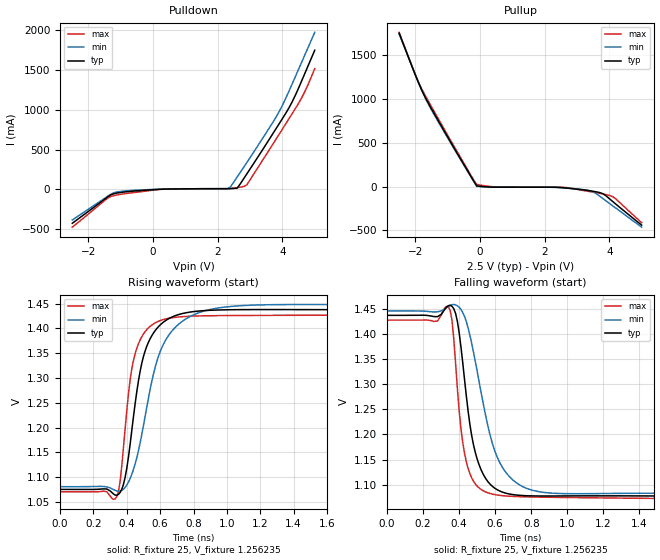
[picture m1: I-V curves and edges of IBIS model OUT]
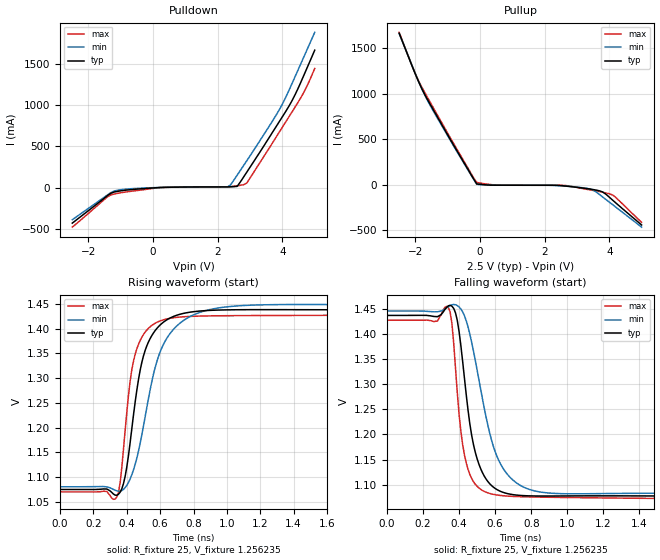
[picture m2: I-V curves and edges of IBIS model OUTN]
|   IBIS File of SG2520VGN D
|   LVDS, Vcc=2.5V, Io=7mA, fo>212.5MHz
[IBIS Ver]   3.2
[File Name]   sg2520vgn_hf_7m_25v.ibs
[File Rev]   1.0
[Date]   July 30, 2020
[Source]
Fairchild Ensigna Lab's Method
[Notes]
Created by Minoru Kozaki
[Disclaimer]
Seiko Epson Corporation makes no warranty with respect to the
information contained herein.
[Copyright]
Copyright(C) 2020, Seiko Epson Corporation. All rights reserved.
|   Component
[Component]   SG2520VGN
[Manufacturer]  Seiko Epson Corporation
[Package]
R_pkg   17.7m   NA   NA
L_pkg   235p   NA   NA
C_pkg   208f   NA   NA
[Pin]   signal_name   model_name   R_pin   L_pin   C_pin
1   OE/ST   NC
2   NC   NC
3   GND   GND
4   OUT   OUT   17.7m   235p   208f
5   OUTN   OUTN   10.4m   129p   221f
6   VCC   POWER
[Diff Pin] inv_pin  vdiff  tdelay_typ
4   5   0   0
| Models and submodels in the file (2): OUT (Output), OUTN (Output)
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|   Model OUT
[Model]   OUT
Model_type   Output
Polarity   Non-Inverting
Vref = 1.25
Vmeas = 1.25
Rref = 25
Cref = 0
C_comp   4.5p   4.5p   4.5p
[Temperature Range]   25   105   -40
[Voltage Range]   2.5   2.25   2.75
[Pullup Reference]   2.5   2.25   2.75
[Pulldown Reference]   0   0   0
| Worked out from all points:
|   slope of the pulldown table from 0 to 0.375 V, typ, clamps not added: 51.8 ohm
|   slope of the pullup table from 0 to 0.375 V, typ, clamps not added: 39.7 ohm
|   falling waveform, R_fixture 25, V_fixture 1.256235: 20-80 % time 89.9ps typ, 138ps min, 65.2ps max; typ from 1.44 V to 1.08 V
|   rising waveform, R_fixture 25, V_fixture 1.256235: 20-80 % time 108ps typ, 157ps min, 81.3ps max; typ from 1.07 V to 1.44 V
[Pullup]
-2.5V     1.75A      1.744A     1.761A
-2V       1.274A     1.28A      1.277A
-1.8V     1.099A     1.1A       1.113A
-1.6V     953.9mA    944mA      977.3mA
-800mV    440.1mA    430.4mA    457.9mA
-100mV    7.335mA    2.483mA    23.32mA
600mV     -6.947mA   -7.059mA   -6.444mA
2.6V      -14.81mA   -15.66mA   -9.067mA
3.4V      -48.22mA   -47.71mA   -57.68mA
3.8V      -81.84mA   -137mA     -84.03mA
4.1V      -168.9mA   -218.5mA   -114mA
5V        -440.6mA   -463.6mA   -412.6mA
[Pulldown]
-2.5V     -426.2mA   -385.4mA   -475.1mA
-1.4V     -92.61mA   -84.86mA   -108mA
-1.2V     -52.56mA   -40.75mA   -76.75mA
300mV     2.535mA    2.627mA    2.312mA
2.3V      8.827mA    8.638mA    9.79mA
2.4V      9.632mA    35.63mA    12.25mA
2.6V      15.06mA    155.9mA    22.1mA
2.9V      195.2mA    338.1mA    57.72mA
3.9V      826.3mA    978.8mA    694.8mA
4.3V      1.1A       1.326A     952.1mA
4.6V      1.37A      1.604A     1.155A
5V        1.751A     1.976A     1.519A
[Falling Waveform]
R_fixture = 25
V_fixture = 1.256235
V_fixture_min = 1.263317
V_fixture_max = 1.249100
0s        1.437V     1.446V     1.428V
340ps     1.456V     1.455V     1.454V
370ps     1.45V      1.459V     1.392V
410ps     1.375V     1.449V     1.212V
450ps     1.246V     1.412V     1.132V
530ps     1.123V     1.268V     1.089V
590ps     1.095V     1.176V     1.081V
660ps     1.083V     1.124V     1.077V
960ps     1.077V     1.082V     1.075V
4ns       1.076V     1.081V     1.071V
[Rising Waveform]
R_fixture = 25
V_fixture = 1.256235
V_fixture_min = 1.263317
V_fixture_max = 1.249100
0s        1.075V     1.081V     1.071V
320ps     1.066V     1.075V     1.055V
360ps     1.069V     1.072V     1.092V
410ps     1.141V     1.09V      1.269V
450ps     1.249V     1.127V     1.349V
520ps     1.364V     1.242V     1.398V
630ps     1.415V     1.375V     1.419V
800ps     1.434V     1.427V     1.425V
1.1ns     1.438V     1.446V     1.426V
4ns       1.437V     1.446V     1.427V
[Ramp]
R_load = 25
dV/dt_r   0.21650/107.63p   0.21785/155.60p   0.21397/80.91p
dV/dt_f   0.21650/89.45p   0.21785/136.75p   0.21397/64.91p
|   Model OUTN
[Model]   OUTN
Model_type   Output
Polarity   Inverting
Vref = 1.25
Vmeas = 1.25
Rref = 25
Cref = 0
C_comp   4.5p   4.5p   4.5p
[Temperature Range]   25   105   -40
[Voltage Range]   2.5   2.25   2.75
[Pullup Reference]   2.5   2.25   2.75
[Pulldown Reference]   0   0   0
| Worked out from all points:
|   slope of the pulldown table from 0 to 0.375 V, typ, clamps not added: 51.8 ohm
|   slope of the pullup table from 0 to 0.375 V, typ, clamps not added: 39.7 ohm
|   falling waveform, R_fixture 25, V_fixture 1.256235: 20-80 % time 89.7ps typ, 137ps min, 65.3ps max; typ from 1.44 V to 1.08 V
|   rising waveform, R_fixture 25, V_fixture 1.256235: 20-80 % time 108ps typ, 157ps min, 81.5ps max; typ from 1.07 V to 1.44 V
[Pullup]
-2.5V     1.665A     1.661A     1.674A
-2V       1.215A     1.22A      1.22A
-1.7V     984.8mA    977.9mA    1.007A
-1V       547.3mA    537.1mA    565.5mA
-100mV    7.335mA    2.486mA    23.28mA
600mV     -6.948mA   -7.061mA   -6.446mA
2.6V      -14.82mA   -15.81mA   -9.069mA
3.4V      -48.75mA   -48.13mA   -58.05mA
3.6V      -61.25mA   -82.56mA   -70.66mA
3.8V      -82.36mA   -137.8mA   -84.8mA
4.1V      -169.9mA   -220.1mA   -114.6mA
5V        -444.2mA   -468mA     -415mA
[Pulldown]
-2.5V     -430.3mA   -389.3mA   -479.1mA
-1.4V     -93.43mA   -85.69mA   -108.6mA
-1.2V     -52.98mA   -41.07mA   -77.28mA
300mV     2.535mA    2.629mA    2.311mA
2.3V      8.828mA    8.639mA    9.791mA
2.4V      9.63mA     34.46mA    12.24mA
2.6V      15.04mA    150.6mA    22.06mA
2.9V      188.5mA    326.4mA    55.94mA
4V        859.3mA    1.013A     732.9mA
4.3V      1.055A     1.264A     919.2mA
4.6V      1.304A     1.529A     1.11A
5V        1.666A     1.882A     1.444A
[Falling Waveform]
R_fixture = 25
V_fixture = 1.256235
V_fixture_min = 1.263317
V_fixture_max = 1.249100
0s        1.437V     1.446V     1.428V
330ps     1.453V     1.452V     1.455V
370ps     1.451V     1.459V     1.381V
410ps     1.376V     1.45V      1.205V
450ps     1.247V     1.414V     1.13V
530ps     1.123V     1.27V      1.088V
590ps     1.095V     1.176V     1.081V
660ps     1.083V     1.124V     1.077V
960ps     1.077V     1.082V     1.075V
4ns       1.076V     1.081V     1.071V
[Rising Waveform]
R_fixture = 25
V_fixture = 1.256235
V_fixture_min = 1.263317
V_fixture_max = 1.249100
0s        1.075V     1.081V     1.071V
330ps     1.064V     1.074V     1.056V
360ps     1.07V      1.072V     1.089V
420ps     1.17V      1.097V     1.294V
450ps     1.252V     1.126V     1.348V
520ps     1.365V     1.241V     1.397V
630ps     1.415V     1.375V     1.418V
800ps     1.434V     1.428V     1.425V
1.1ns     1.438V     1.446V     1.426V
4ns       1.437V     1.446V     1.427V
[Ramp]
R_load = 25
dV/dt_r   0.21619/107.45p  0.21803/155.27p  0.21366/81.06p
dV/dt_f   0.21619/89.12p   0.21803/136.08p  0.21366/64.90p
